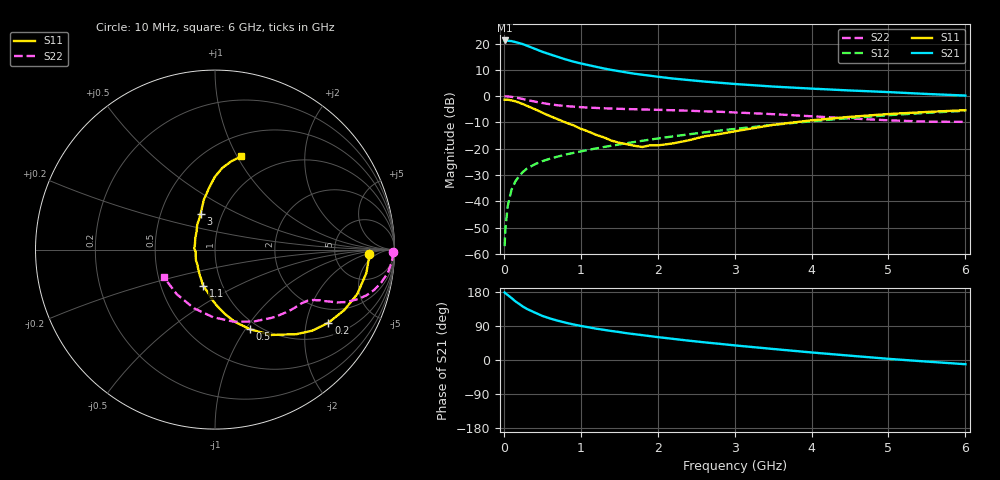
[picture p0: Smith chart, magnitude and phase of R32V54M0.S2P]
! SIEMENS Small Signal Semiconductors
! BFR181
! Si NPN RF Bipolar Junction Transistor in SOT23
! VCE = 2.5 V  IC = 4 mA
! Common Emitter S-Parameters:  May  1996
# GHz  S  MA  R  50
!  f  S11  S21  S12  S22
! GHz  MAG  ANG  MAG  ANG  MAG  ANG  MAG  ANG
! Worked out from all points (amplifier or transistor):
!   36 points, 10 MHz to 6 GHz, reference 50 ohm
!   highest |S21| = 21.2 dB at 10 MHz (marker M1)
!   |S21| within 3 dB of that: start of sweep to 387.5 MHz
!   unconditionally stable (mu >= 1): 1.202 GHz to 3.092 GHz
!   at 250 MHz: K = 0.37, MSG = 24.3 dB, |S12| = -28.8 dB
!   at 1.4 GHz: K = 1.04, MAG = 13.2 dB, |S12| = -18.9 dB
!   at 6 GHz: K = 0.86, MSG = 2.9 dB, |S12| = -5.6 dB
!   S11 on the Smith chart (normalised r, x): 10 MHz: 13, -3; 200 MHz: 1.44, -2.70; 500 MHz: 0.91, -1.05; 1.1 GHz: 0.81, -0.34; 3 GHz: 0.79, +0.33; 6 GHz: 0.71, +1.04
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0.01  0.8584 -1.8  11.48 178.3  0.0014 93.0  0.9937 -0.8
0.02  0.8583 -3.5  11.48 176.3  0.003 86.1  0.9926 -1.7
0.05  0.8533 -8.8  11.34 171.6  0.0081 84.9  0.9874 -4.0
0.1  0.8307 -17.3  11.15 163.5  0.0166 80.7  0.971 -7.8
0.15  0.7957 -25.0  10.71 154.8  0.0239 76.2  0.9426 -11.4
0.2  0.752 -32.8  10.22 147.9  0.0303 72.9  0.9139 -14.3
0.25  0.7056 -39.8  9.737 140.8  0.0364 69.7  0.8813 -16.8
0.3  0.6539 -46.1  9.121 134.8  0.0418 67.7  0.8473 -18.9
0.4  0.5684 -56.8  7.991 125.5  0.0504 64.2  0.7894 -21.7
0.5  0.4845 -66.3  6.991 116.4  0.058 62.2  0.7411 -23.4
0.6  0.4175 -74.6  6.249 109.6  0.0645 61.3  0.7006 -24.4
0.7  0.3644 -81.0  5.597 103.8  0.0709 61.0  0.6711 -25.3
0.8  0.3168 -87.5  5.017 98.6  0.0773 60.6  0.6485 -25.8
0.9  0.2806 -93.1  4.558 94.0  0.083 60.7  0.6324 -26.5
1.1  0.212 -108.2  3.895 86.4  0.0952 61.4  0.6061 -27.7
1.6  0.1218 -150.4  2.816 70.6  0.1277 62.2  0.569 -31.6
2.2  0.1264 150.4  2.163 55.8  0.1718 61.4  0.5391 -38.7
3  0.2141 112.1  1.706 38.6  0.2381 57.5  0.4904 -51.2
3.5  0.2847 102.6  1.523 29.1  0.2841 53.8  0.4546 -61.9
4.5  0.4045 90.2  1.283 11.4  0.384 43.8  0.3769 -91.6
5.5  0.5006 79.5  1.101 -4.2  0.482 31.2  0.3273 -130.7
6  0.5412 74.2  1.027 -11.1  0.5265 24.1  0.3242 -152.0
